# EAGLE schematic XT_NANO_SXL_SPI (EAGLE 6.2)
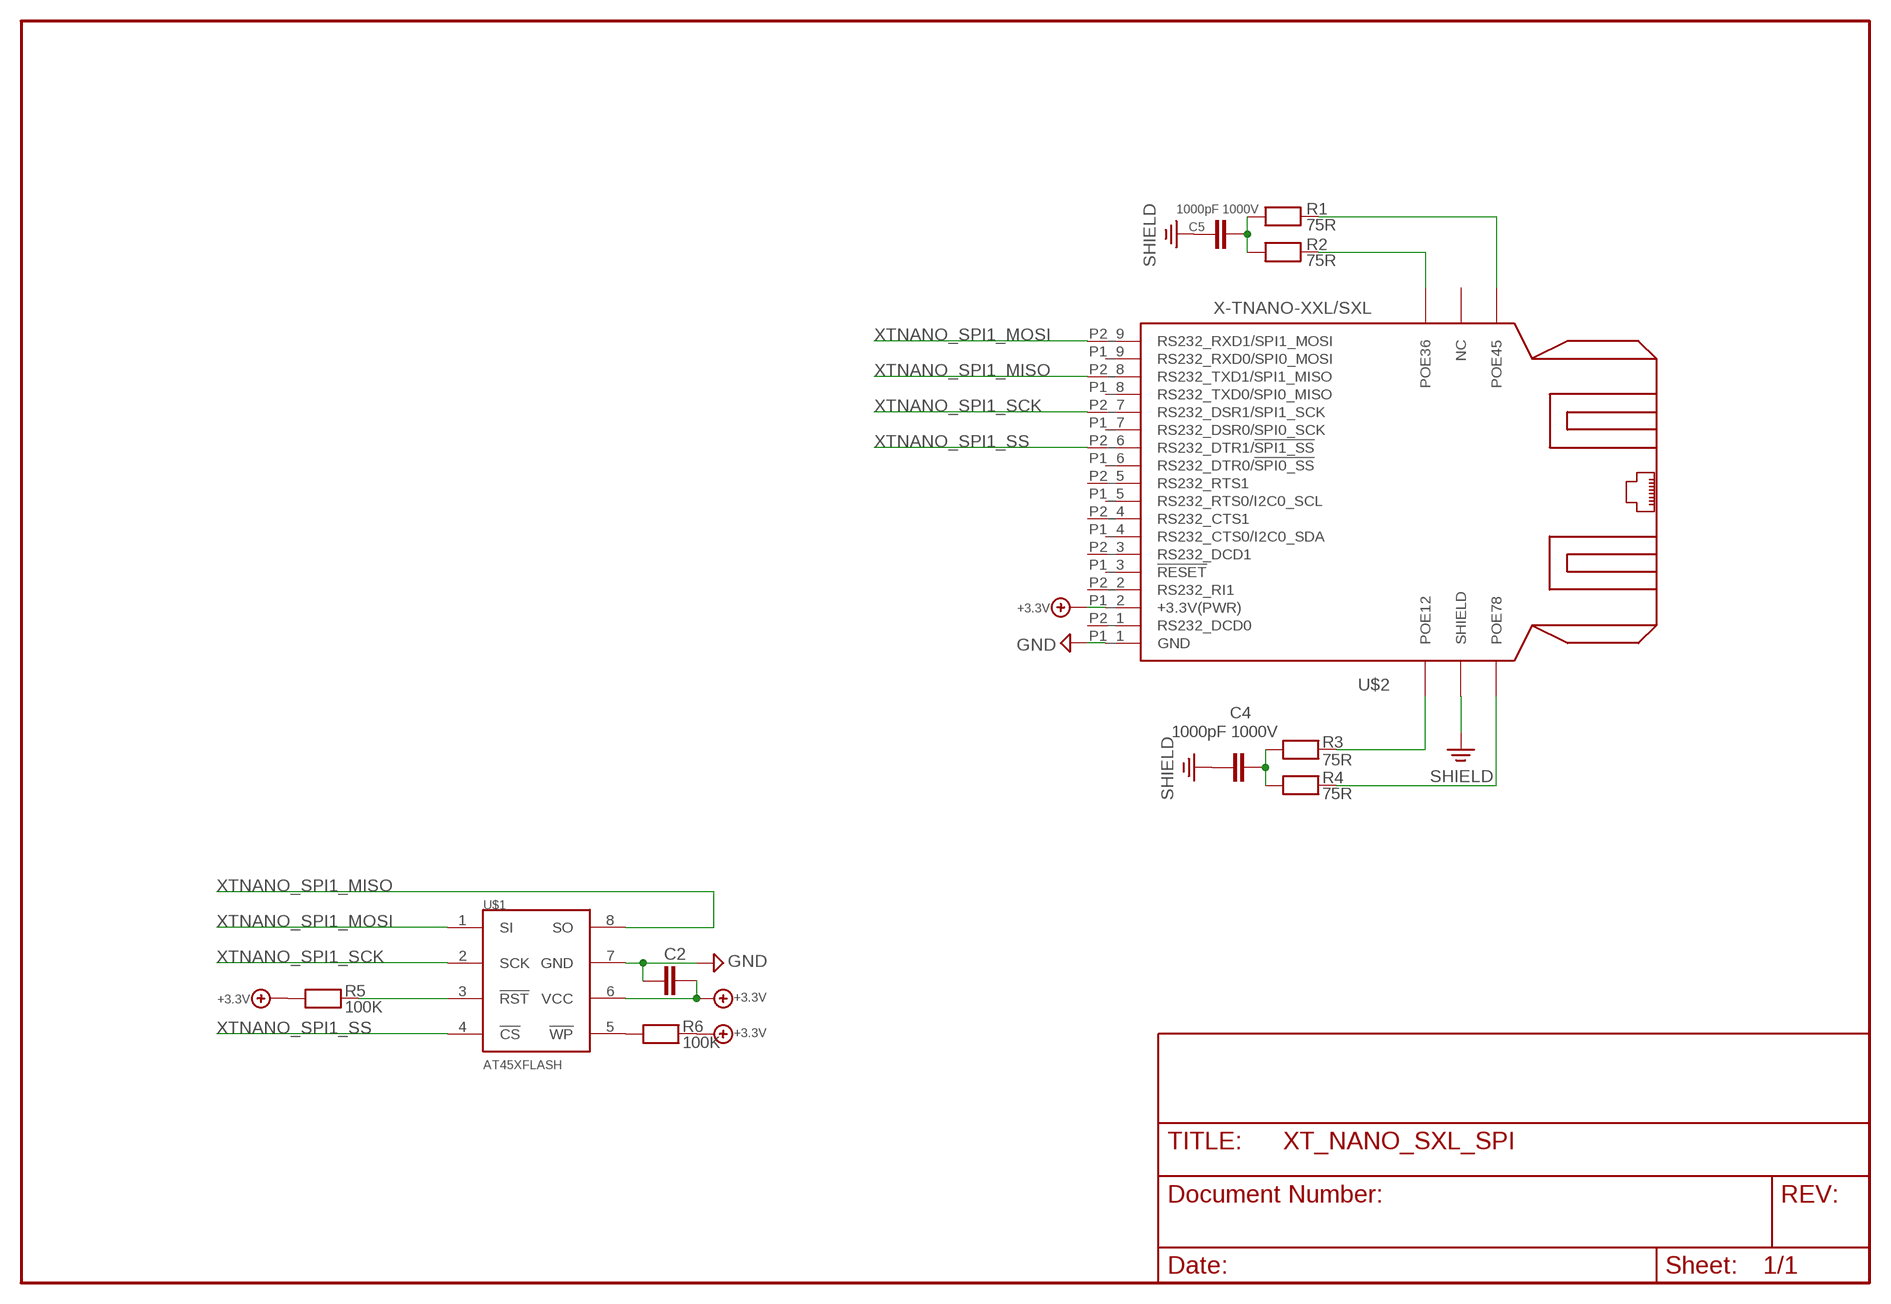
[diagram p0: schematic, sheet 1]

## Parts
C2  CHIP-C-0805  [SMD-0805]
C4  1000pF 1000V  CHIP-C-1210  [SMD-1210]
C5  1000pF 1000V  CHIP-C-1210  [SMD-1210]
R1  75R  CHIP-R-0603  [SMD-0603]
R2  75R  CHIP-R-0603  [SMD-0603]
R3  75R  CHIP-R-0603  [SMD-0603]
R4  75R  CHIP-R-0603  [SMD-0603]
R5  100K  CHIP-R-0603  [SMD-0603]
R6  100K  CHIP-R-0603  [SMD-0603]
U$1  AT45XFLASH  [SO-8]
U$2  X-TNANO-XXL/SXL  [XT-NANO-XXL/SXL]

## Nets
+3.3V: C2.2 R5.1 R6.2 U$1.6(VCC) U$2.P1_2(+3.3V(PWR))
GND: C2.1 U$1.7(GND) U$2.P1_1(GND)
N$1: C5.1 R1.1 R2.1
N$2: C4.2 R3.1 R4.1
N$3: R5.2 U$1.3(!RST)
N$4: R2.2 U$2.POE36
N$5: R6.1 U$1.5(!WP)
N$6: R1.2 U$2.POE45
N$20: R3.2 U$2.POE12
N$21: R4.2 U$2.POE78
SHIELD: C4.1 C5.2 U$2.SHIELD
XTNANO_SPI1_MISO: U$1.8(SO) U$2.P2_8(RS232_TXD1/SPI1_MISO)
XTNANO_SPI1_MOSI: U$1.1(SI) U$2.P2_9(RS232_RXD1/SPI1_MOSI)
XTNANO_SPI1_SCK: U$1.2(SCK) U$2.P2_7(RS232_DSR1/SPI1_SCK)
XTNANO_SPI1_SS: U$1.4(!CS) U$2.P2_6(RS232_DTR1/!SPI1_SS!)
Unconnected: U$2.FLASH(NC) U$2.P1_3(!RESET) U$2.P1_4(RS232_CTS0/I2C0_SDA) U$2.P1_5(RS232_RTS0/I2C0_SCL) U$2.P1_6(RS232_DTR0/!SPI0_SS!) U$2.P1_7(RS232_DSR0/SPI0_SCK) U$2.P1_8(RS232_TXD0/SPI0_MISO) U$2.P1_9(RS232_RXD0/SPI0_MOSI) U$2.P2_1(RS232_DCD0) U$2.P2_2(RS232_RI1) U$2.P2_3(RS232_DCD1) U$2.P2_4(RS232_CTS1) U$2.P2_5(RS232_RTS1)

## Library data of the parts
C2 C4 C5 = XTMACRO:CHIP-C-?: Chip capacitance
R1-R6 = XTMACRO:CHIP-R-?: Chip resistors
U$1 = xtnano:AT45XFLASH
U$2 = ak-devices:X-TNANO-XXL/SXL: AK-NORD XT-NANO-XXL/SXL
